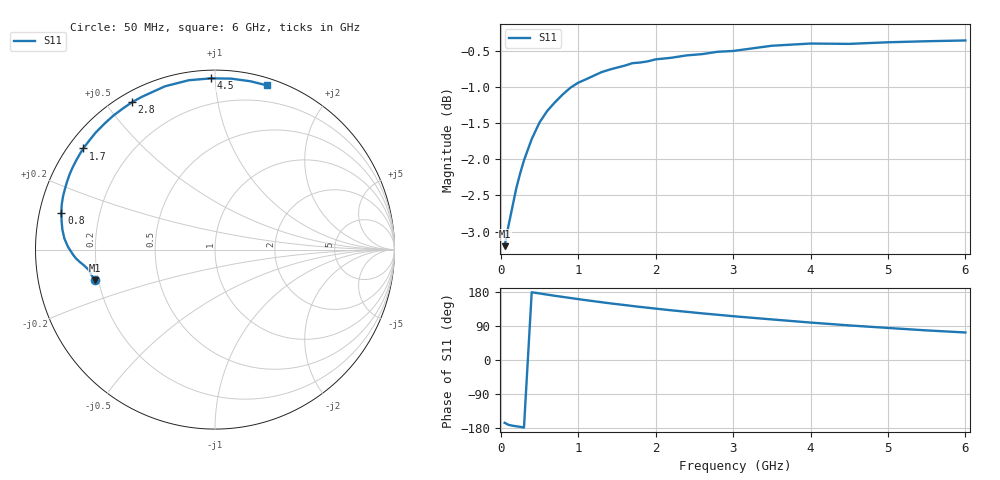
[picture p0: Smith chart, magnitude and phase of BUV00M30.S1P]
! Infineon Technologies  Discrete & RF Semiconductors
! BB 833
! Si Tuning Diode in SOD323
! VR =
! S-Parameters:  June  1999
# GHz  S  MA  R  50
!  f  S11
! GHz  MAG  ANG
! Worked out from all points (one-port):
!   34 points, 50 MHz to 6 GHz, reference 50 ohm
!   lowest |S11| = -3.2 dB at 50 MHz (marker M1), VSWR 5.49, Z = 9.25 - j6.06 ohm
!   |S11| at or under -10 dB: nowhere
!   S11 on the Smith chart (normalised r, x): 50 MHz: 0.19, -0.12; 800 MHz: 0.06, +0.12; 1.7 GHz: 0.04, +0.34; 2.8 GHz: 0.04, +0.58; 4.5 GHz: 0.05, +0.98; 6 GHz: 0.06, +1.36
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0.05  0.6917 -165.7
0.1  0.7145 -171.1
0.15  0.736 -173.2
0.2  0.7582 -174.9
0.25  0.7764 -176.4
0.3  0.7928 -178.1
0.4  0.8202 178.8
0.5  0.842 175.7
0.6  0.8577 172.5
0.8  0.8805 166.5
0.9  0.8901 163.6
1  0.8972 160.7
1.2  0.9072 155.2
1.4  0.9159 149.9
1.6  0.9218 145.0
1.7  0.9255 142.5
2  0.9312 135.6
2.2  0.9335 131.2
2.4  0.937 127.2
2.6  0.9389 123.1
2.8  0.9425 119.4
3  0.9436 115.6
3.5  0.9515 107.1
4  0.9549 98.8
4.5  0.9544 91.3
5  0.9568 84.6
5.5  0.9584 78.1
6  0.9596 72.6
